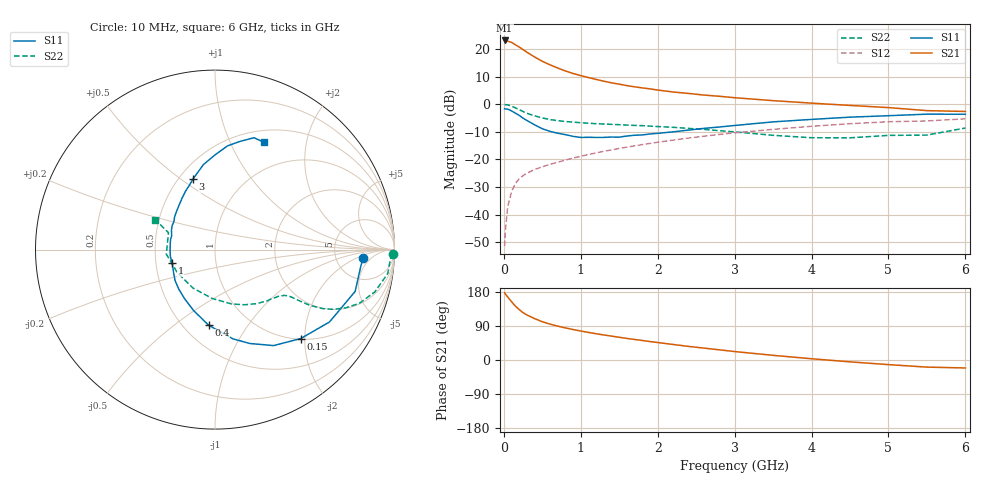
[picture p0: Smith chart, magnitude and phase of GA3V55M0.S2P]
! Infineon Technologies  Discrete & RF Semiconductors
! BF775
! Si NPN RF Bipolar Junction Transistor in SOT23
! VCE = 3.5 V  IC = 5 mA
! Common Emitter S-Parameters:  May  1996
# GHz  S  MA  R  50
!  f  S11  S21  S12  S22
! GHz  MAG  ANG  MAG  ANG  MAG  ANG  MAG  ANG
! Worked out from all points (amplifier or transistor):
!   36 points, 10 MHz to 6 GHz, reference 50 ohm
!   highest |S21| = 23.1 dB at 10 MHz (marker M1)
!   |S21| within 3 dB of that: start of sweep to 233.6 MHz
!   unconditionally stable (mu >= 1): 797.1 MHz to 3.406 GHz
!   at 250 MHz: K = 0.49, MSG = 22.8 dB, |S12| = -25.9 dB
!   at 1.4 GHz: K = 1.12, MAG = 10.0 dB, |S12| = -16.5 dB
!   at 6 GHz: K = 0.96, MSG = 1.3 dB, |S12| = -5.3 dB
!   lowest NFmin = 1.50 dB at 450 MHz
!   S11 on the Smith chart (normalised r, x): 10 MHz: 10, -3; 150 MHz: 1.02, -1.91; 400 MHz: 0.66, -0.67; 1 GHz: 0.61, -0.10; 3 GHz: 0.59, +0.55; 6 GHz: 0.64, +1.35
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0.01  0.8262 -3.4  14.21 177.2  0.0027 87.1  0.9918 -1.4
0.02  0.8174 -6.6  14.02 174.2  0.0052 86.1  0.9785 -3.2
0.05  0.815 -16.6  13.8 166.4  0.0139 81.6  0.9717 -7.9
0.1  0.7546 -32.3  13.13 153.8  0.0261 72.6  0.9213 -14.8
0.15  0.6886 -46.0  11.87 142.2  0.0366 67.6  0.8583 -20.4
0.2  0.6266 -58.6  10.81 133.0  0.0448 63.5  0.7961 -24.1
0.25  0.5577 -69.7  9.709 124.9  0.0508 59.8  0.7352 -26.9
0.3  0.5074 -78.6  8.701 118.8  0.0565 58.2  0.6849 -28.7
0.4  0.4228 -94.8  7.137 109.3  0.0657 56.1  0.6151 -30.4
0.5  0.36 -109.3  5.965 101.0  0.0739 55.8  0.5636 -31.1
0.6  0.3222 -121.6  5.149 94.7  0.0815 56.1  0.5271 -31.5
0.8  0.281 -142.6  3.99 84.7  0.0974 56.6  0.4856 -32.2
1  0.2503 -162.7  3.286 76.5  0.114 57.2  0.4622 -33.5
1.1  0.2516 -171.2  3.03 72.8  0.1229 57.5  0.4524 -34.7
1.3  0.2508 174.2  2.602 66.1  0.1405 57.5  0.4369 -36.7
1.6  0.2655 156.1  2.165 56.9  0.1671 56.6  0.4179 -40.8
2.2  0.3158 129.8  1.661 41.0  0.2238 53.0  0.3819 -52.0
3  0.4117 107.4  1.309 22.3  0.3029 45.3  0.3157 -73.3
3.5  0.4786 97.7  1.158 12.3  0.3501 39.5  0.2733 -92.9
4.5  0.5822 83.1  0.949 -4.9  0.4431 26.6  0.2462 -148.3
5.5  0.66 70.8  0.764 -18.8  0.4974 11.6  0.2758 160.0
6  0.6572 65.5  0.738 -21.0  0.543 7.4  0.3705 153.5
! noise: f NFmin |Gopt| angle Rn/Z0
0.45  1.5  0.28  29  0.34
0.9  1.8  0.25  59  0.34
